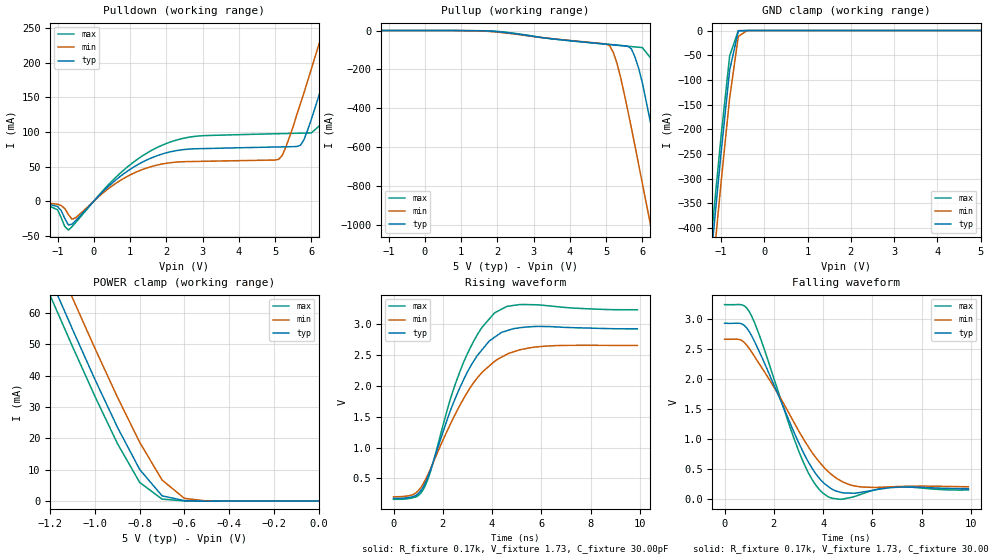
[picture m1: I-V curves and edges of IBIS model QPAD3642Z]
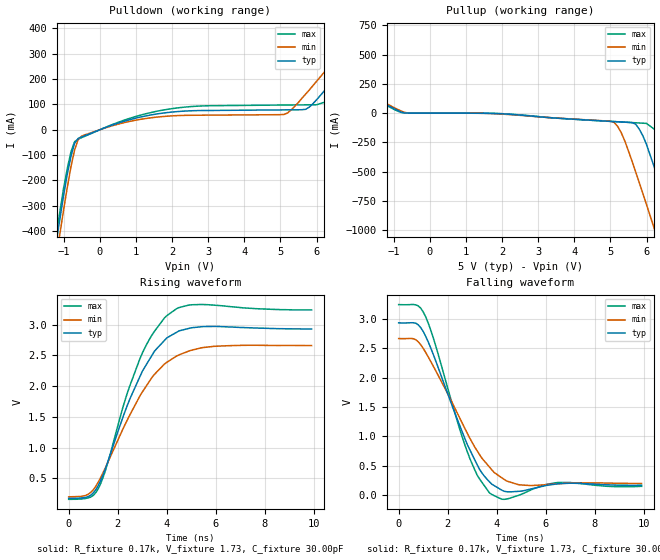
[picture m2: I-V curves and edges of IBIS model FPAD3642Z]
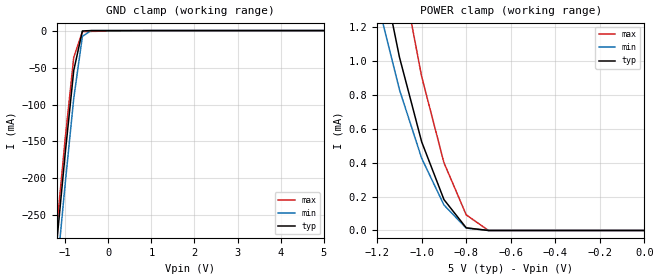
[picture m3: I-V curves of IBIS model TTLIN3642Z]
| IBIS file 723622.ibs created by s2ibis2 version 1.1
| North Carolina State University Electronics Research Laboratory  1995
[IBIS ver]   2.1
[File name]   723622.ibs
[File Rev]   1.0
[Date]   08/22/97
[Source]   Integrated Device Technology, Inc.
[Notes]   1. Temperatures: typ=25C, min=70C, max=0C 2. Cemos7_5v
   process. 3. Ramp rates based on 50 ohm load.
[Copyright]   Copyright 1997, Integrated Device Technology, Inc.
|   Component idt723622
[Component]   idt723622
[Manufacturer]   Integrated Device Technology
[Package]
| variable   typ   min   max
R_pkg   0.75   0.60   0.90
L_pkg   8.10nH   8.30nH   9.90nH
C_pkg   0.53pF   0.46pF   0.60pF
[Pin]  signal_name   model_name   R_pin   L_pin   C_pin
1   A35   QPAD3642Z
2   A34   QPAD3642Z
3   A33   QPAD3642Z
4   A32   QPAD3642Z
5   VCC   POWER
6   A31   QPAD3642Z
7   A30   QPAD3642Z
8   GND   GND
9   A29   QPAD3642Z
10   A28   QPAD3642Z
11   A27   QPAD3642Z
12   A26   QPAD3642Z
13   A25   QPAD3642Z
14   A24   QPAD3642Z
15   A23   QPAD3642Z
16   GND   GND
17   A22   QPAD3642Z
18   VCC   POWER
19   A21   QPAD3642Z
20   A20   QPAD3642Z
21   A19   QPAD3642Z
22   A18   QPAD3642Z
23   GND   GND
24   A17   QPAD3642Z
25   A16   QPAD3642Z
26   A15   QPAD3642Z
27   A14   QPAD3642Z
28   A13   QPAD3642Z
29   VCC   POWER
30   A12   QPAD3642Z
31   GND   GND
32   A11   QPAD3642Z
33   A10   QPAD3642Z
34   A9   QPAD3642Z
35   A8   QPAD3642Z
36   A7   QPAD3642Z
37   A6   QPAD3642Z
38   GND   GND
39   A5   QPAD3642Z
40   A4   QPAD3642Z
41   A3   QPAD3642Z
42   VCC   POWER
43   A2   QPAD3642Z
44   A1   QPAD3642Z
45   A0   QPAD3642Z
46   GND   GND
47   B0   QPAD3642Z
48   B1   QPAD3642Z
49   B2   QPAD3642Z
50   B3   QPAD3642Z
51   B4   QPAD3642Z
52   B5   QPAD3642Z
53   GND   GND
54   B6   QPAD3642Z
55   VCC   POWER
56   B7   QPAD3642Z
57   B8   QPAD3642Z
58   B9   QPAD3642Z
59   B10   QPAD3642Z
60   B11   QPAD3642Z
61   GND   GND
62   B12   QPAD3642Z
63   B13   QPAD3642Z
64   B14   QPAD3642Z
65   B15   QPAD3642Z
66   VCC   POWER
67   B16   QPAD3642Z
68   B17   QPAD3642Z
69   GND   GND
70   B18   QPAD3642Z
71   B19   QPAD3642Z
72   B20   QPAD3642Z
73   B21   QPAD3642Z
74   B22   QPAD3642Z
75   B23   QPAD3642Z
76   GND   GND
77   B24   QPAD3642Z
78   B25   QPAD3642Z
79   VCC   POWER
80   B26   QPAD3642Z
81   B27   QPAD3642Z
82   B28   QPAD3642Z
83   B29   QPAD3642Z
84   B30   QPAD3642Z
85   B31   QPAD3642Z
86   GND   GND
87   B32   QPAD3642Z
88   B33   QPAD3642Z
89   B34   QPAD3642Z
90   B35   QPAD3642Z
91   VCC   POWER
92   CLKB   TTLIN3642Z
93   ENB   TTLIN3642Z
94   W_RB   TTLIN3642Z
95   CSBL   TTLIN3642Z
96   GND   GND
97   IRB   FPAD3642Z
98   ORB   FPAD3642Z
99   AFBL   FPAD3642Z
100   AEBL   FPAD3642Z
101   VCC   POWER
102   MBF1   FPAD3642Z
103   MBB   TTLIN3642Z
104   RST2   TTLIN3642Z
105   FS1   TTLIN3642Z
106   GND   GND
107   FS0   TTLIN3642Z
108   RST1   TTLIN3642Z
109   MBA   TTLIN3642Z
110   MBF2   FPAD3642Z
111   AEAL   FPAD3642Z
112   AFAL   FPAD3642Z
113   VCC   POWER
114   ORA   FPAD3642Z
115   IRA   FPAD3642Z
116   CSAL   TTLIN3642Z
117   W_RA   TTLIN3642Z
118   ENA   TTLIN3642Z
119   CLKA   TTLIN3642Z
120   GND   GND
| Models and submodels in the file (3): QPAD3642Z (I/O), FPAD3642Z (Output), TTLIN3642Z (Input)
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| FIN  FIN   dummy_model
| QIN  QIN   dummy_model
| QOEL QOEL   dummy_model
|   Model QPAD3642Z
[Model]   QPAD3642Z
Model_type   I/O
Polarity   Non-Inverting
Enable   Active-Low
Vinl =  0.000V
Vinh =  3.000V
Vmeas =  1.500V
C_comp   3.00pF   NA   NA
[Temperature Range]   25.00   70.00   0.000
[Voltage Range]   5.00V   4.50V   5.50V
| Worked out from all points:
|   slope of the pulldown table from 0 to 0.75 V, typ, clamps not added: 20.5 ohm
|   slope of the pullup table from 0 to 0.75 V, typ, clamps not added: 25.9 kohm
|   GND clamp passes 1 mA (typ) near -0.60 V on its own axis
|   POWER clamp passes 1 mA (typ) near -0.66 V on its own axis
|   rising waveform, R_fixture 0.17k, V_fixture 1.73, C_fixture 30.00pF: 20-80 % time 1.64ns typ, 1.93ns min, 1.5ns max; typ from 0.176 V to 2.93 V
|   falling waveform, R_fixture 0.17k, V_fixture 1.73, C_fixture 30.00pF: 20-80 % time 1.77ns typ, 2.16ns min, 1.53ns max; typ from 2.93 V to 0.173 V
[Pulldown]
| voltage   I(typ)   I(min)   I(max)
-5V       0A         -1mA       0A
-1.4V     -2.6mA     -1.9mA     -3.1mA
-1V       -7.7mA     -4.4mA     -12.4mA
-700mV    -34.39mA   -19.37mA   -41.73mA
700mV     34.57mA    28.94mA    39.05mA
1.8V      66.7mA     52.82mA    78.9mA
5.1V      78.42mA    60.43mA    97.58mA
5.7V      80.72mA    141mA      98.3mA
6.4V      184mA      259mA      117mA
6.8V      252mA      327mA      181mA
7.2V      320mA      396mA      249mA
10V       806mA      882mA      734mA
[Pullup]
| voltage   I(typ)   I(min)   I(max)
-5V       0A         0A         0A
1.8V      -3.202mA   -5.178mA   -2.04mA
5V        -69.89mA   -69.05mA   -70.44mA
5.1V      -71.61mA   -78.32mA   -72.17mA
5.3V      -75.05mA   -168mA     -75.61mA
5.7V      -94.45mA   -503mA     -82.44mA
6V        -268mA     -784mA     -87.54mA
6.4V      -630mA     -1.165A    -181mA
6.8V      -1.01A     -1.55A     -504mA
7.2V      -1.395A    -1.938A    -882mA
7.6V      -1.782A    -2.326A    -1.266A
10V       -4.125A    -4.67A     -3.606A
[GND_clamp]
| voltage   I(typ)   I(min)   I(max)
-5V       -4.123A    -4.179A    -4.092A
-1.4V     -620mA     -681mA     -587mA
-1.2V     -432mA     -493mA     -398mA
-1V       -249mA     -309mA     -215mA
-800mV    -80.04mA   -136mA     -51.24mA
-600mV    -972uA     -12mA      -154uA
-400mV    -331nA     -19.33uA   -23.45nA
5V        50nA       49.06uA    50nA
[POWER_clamp]
| voltage   I(typ)   I(min)   I(max)
-5V       723mA      732mA      718mA
-1.2V     70.9mA     80.87mA    65.4mA
-1.1V     54.63mA    64.6mA     49.14mA
-1V       38.73mA    48.62mA    33.34mA
-900mV    23.59mA    33.19mA    18.39mA
-800mV    10.08mA    18.74mA    5.951mA
-700mV    1.694mA    6.736mA    642uA
-600mV    151uA      876uA      70.05uA
-500mV    817nA      49.07uA    125nA
0V        50nA       45.12nA    55nA
[Ramp]
| variable   typ   min   max
dV/dt_r   1.07/0.80n   0.91/1.01n   1.23/0.70n
dV/dt_f   1.94/2.25n   1.56/2.83n   2.27/1.87n
R_load = 50.00
[Rising Waveform]
R_fixture = 0.17k
V_fixture = 1.73
C_fixture = 30.00pF
R_dut = 0.75
L_dut = 8.10nH
C_dut = 0.53pF
| time   V(typ)   V(min)   V(max)
0s        176mV      201mV      161mV
800ps     207mV      240mV      188mV
1.2ns     357mV      409mV      315mV
1.5ns     637mV      654mV      610mV
2.3ns     1.592V     1.374V     1.778V
2.8ns     2.064V     1.763V     2.343V
3.5ns     2.543V     2.179V     2.896V
4.1ns     2.791V     2.399V     3.185V
5.7ns     2.965V     2.63V      3.319V
9.9ns     2.928V     2.658V     3.237V
[Falling Waveform]
R_fixture = 0.17k
V_fixture = 1.73
C_fixture = 30.00pF
R_dut = 0.75
L_dut = 8.10nH
C_dut = 0.53pF
| time   V(typ)   V(min)   V(max)
0s        2.931V     2.664V     3.241V
600ps     2.93V      2.66V      3.243V
1ns       2.793V     2.511V     3.127V
1.5ns     2.377V     2.197V     2.632V
3.1ns     862mV      1.073V     710mV
4ns       280mV      546mV      98.93mV
4.7ns     114mV      310mV      -3.433mV
5.5ns     111mV      205mV      75.17mV
7ns       197mV      209mV      208mV
9.9ns     173mV      206mV      152mV
|   Model FPAD3642Z
[Model]   FPAD3642Z
Model_type   Output
Vmeas =  1.500V
C_comp   3.00pF   NA   NA
[Temperature Range]   25.00   70.00   0.000
[Voltage Range]   5.00V   4.50V   5.50V
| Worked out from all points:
|   slope of the pulldown table from 0 to 0.75 V, typ, clamps not added: 20.5 ohm
|   slope of the pullup table from 0 to 0.75 V, typ, clamps not added: 25.8 kohm
|   rising waveform, R_fixture 0.17k, V_fixture 1.73, C_fixture 30.00pF: 20-80 % time 1.65ns typ, 1.93ns min, 1.5ns max; typ from 0.176 V to 2.93 V
|   falling waveform, R_fixture 0.17k, V_fixture 1.73, C_fixture 30.00pF: 20-80 % time 1.54ns typ, 1.85ns min, 1.32ns max; typ from 2.93 V to 0.171 V
[Pulldown]
| voltage   I(typ)   I(min)   I(max)
-5V       -4.111A    -4.167A    -4.08A
-1.4V     -621mA     -681mA     -588mA
-1V       -255mA     -313mA     -227mA
-700mV    -53.07mA   -80.18mA   -47.24mA
-500mV    -28.01mA   -24.68mA   -30.93mA
1.9V      68.38mA    53.88mA    81.24mA
5.1V      78.42mA    60.43mA    97.58mA
5.7V      80.72mA    141mA      98.3mA
6.4V      184mA      259mA      117mA
7.6V      389mA      465mA      318mA
8.4V      528mA      604mA      456mA
10V       806mA      882mA      734mA
[Pullup]
| voltage   I(typ)   I(min)   I(max)
-5V       723mA      732mA      718mA
-800mV    10.08mA    18.74mA    5.951mA
1.9V      -4.537mA   -6.706mA   -3.085mA
5.1V      -71.61mA   -78.19mA   -72.17mA
5.3V      -75.05mA   -167mA     -75.61mA
5.7V      -94.3mA    -502mA     -82.44mA
6V        -268mA     -781mA     -87.54mA
6.4V      -628mA     -1.161A    -180mA
6.8V      -1.006A    -1.545A    -502mA
7.2V      -1.391A    -1.931A    -879mA
7.6V      -1.777A    -2.319A    -1.262A
10V       -4.112A    -4.655A    -3.595A
[Ramp]
| variable   typ   min   max
dV/dt_r   1.07/0.84n   0.91/1.03n   1.23/0.72n
dV/dt_f   1.96/1.74n   1.59/2.21n   2.28/1.43n
R_load = 50.00
[Rising Waveform]
R_fixture = 0.17k
V_fixture = 1.73
C_fixture = 30.00pF
R_dut = 0.75
L_dut = 8.10nH
C_dut = 0.53pF
| time   V(typ)   V(min)   V(max)
0s        176mV      201mV      161mV
800ps     206mV      244mV      184mV
1.2ns     380mV      435mV      330mV
1.5ns     661mV      677mV      631mV
2.4ns     1.697V     1.459V     1.899V
2.9ns     2.151V     1.838V     2.441V
3.5ns     2.569V     2.192V     2.891V
4ns       2.783V     2.387V     3.143V
5.5ns     2.967V     2.627V     3.324V
9.9ns     2.927V     2.658V     3.237V
[Falling Waveform]
R_fixture = 0.17k
V_fixture = 1.73
C_fixture = 30.00pF
R_dut = 0.75
L_dut = 8.10nH
C_dut = 0.53pF
| time   V(typ)   V(min)   V(max)
0s        2.931V     2.664V     3.241V
700ps     2.924V     2.643V     3.237V
1.1ns     2.703V     2.429V     3.034V
2.8ns     860mV      1.052V     737mV
3.2ns     517mV      754mV      341mV
3.7ns     228mV      480mV      40.98mV
4.2ns     88.14mV    299mV      -66.74mV
4.9ns     68mV       179mV      1.264mV
6.5ns     196mV      196mV      218mV
9.9ns     171mV      201mV      152mV
|   Model TTLIN3642Z
[Model]   TTLIN3642Z
Model_type   Input
Vinl =  0.000V
Vinh =  3.000V
Vmeas =  1.500V
C_comp   3.00pF   NA   NA
[Temperature Range]   25.00   70.00   0.000
[Voltage Range]   5.00V   4.50V   5.50V
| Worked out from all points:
|   GND clamp passes 1 mA (typ) near -0.60 V on its own axis
|   POWER clamp passes 1 mA (typ) near -1.10 V on its own axis
[GND_clamp]
| voltage   I(typ)   I(min)   I(max)
-5V       -2.772A    -2.809A    -2.759A
-1.2V     -290mA     -331mA     -270mA
-1V       -167mA     -208mA     -147mA
-800mV    -53.79mA   -91.48mA   -36.1mA
-600mV    -517uA     -7.891mA   -1.465mA
-400mV    -227nA     -13.17uA   -1.116mA
800mV     8nA        8.01nA     -40.1uA
5V        50nA       50.09nA    50nA
[POWER_clamp]
| voltage   I(typ)   I(min)   I(max)
-5V       69.72mA    59.04mA    81mA
-1.2V     1.67mA     1.357mA    2.454mA
-1.1V     1.022mA    830uA      1.596mA
-1V       522uA      425uA      906uA
-900mV    182uA      150uA      399uA
-800mV    15.59uA    13.98uA    92.07uA
-700mV    57nA       52.09nA    62nA
0V        50nA       45.08nA    55nA
